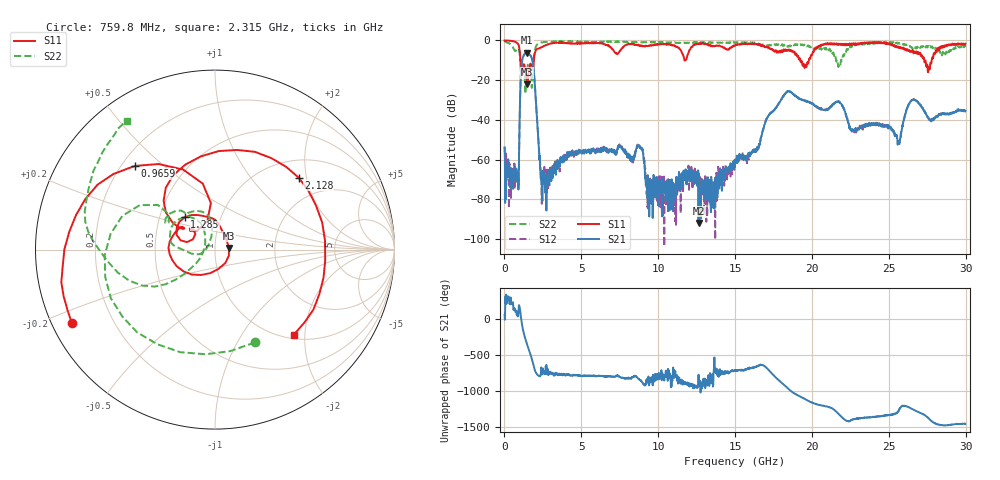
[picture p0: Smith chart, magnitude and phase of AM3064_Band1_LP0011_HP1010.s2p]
# Hz S DB R 50.0
!freq dBS11 angS11 dBS21 angS21 dBS12 angS12 dBS22 angS22
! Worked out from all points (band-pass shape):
!   1600 points, 10 MHz to 29.98 GHz, reference 50 ohm
!   highest |S21| = -6.19 dB at 1.453 GHz (marker M1); lowest = -92.0 dB at 12.62 GHz (marker M2)
!   |S21| within 3 dB of the highest: 1.175 GHz to 1.787 GHz (612 MHz wide, 41.3 % of centre)
!   lowest |S11| = -22.1 dB at 1.491 GHz (marker M3), VSWR 1.17, Z = 58.4 + j0.987 ohm
!   |S11| at or under -10 dB: 1.031 GHz to 1.914 GHz (882.9 MHz wide, 60 % of centre); 19.25 GHz to 19.81 GHz (557.6 MHz wide, 2.86 % of centre); 27.3 GHz to 27.79 GHz (490.7 MHz wide, 1.78 % of centre)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
!   |S22| runs from -26.9 to -0.2 dB; largest |S21 - S12| = 0.0086
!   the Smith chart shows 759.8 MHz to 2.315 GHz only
!   S11 on the Smith chart (normalised r, x): 759.8 MHz: 0.06, -0.24; 965.9 MHz: 0.25, +0.40; 1.285 GHz: 0.67, +0.26; 2.128 GHz: 1.39, +1.80; 2.315 GHz: 1.08, -1.76
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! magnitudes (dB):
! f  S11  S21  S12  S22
! 10 MHz  -0.1  -53.9  -53.5  -0.2
! 759.8 MHz  -0.9  -65.1  -65.3  -5.0
! 965.9 MHz  -3.8  -49.3  -49.2  -5.2
! 1.285 GHz  -12.2  -7.2  -7.1  -14.2
! 1.453 GHz  -20.0  -6.2  -6.1  -15.9
! 1.491 GHz  -22.1  -6.3  -6.2  -13.5
! 1.828 GHz  -13.4  -10.5  -10.4  -17.7
! 2.128 GHz  -4.2  -40.6  -40.2  -2.2
! 2.315 GHz  -3.8  -64.8  -59.9  -1.2
! 5.015 GHz  -1.5  -56.2  -56.3  -0.8
! 8.801 GHz  -2.7  -53.5  -54.0  -0.9
! 9.326 GHz  -2.9  -67.8  -73.4  -1.0
! 10 GHz  -2.0  -70.9  -79.6  -0.9
! 12.62 GHz  -1.6  -92.0  -70.1  -0.9
! 15 GHz  -2.5  -62.1  -60.8  -1.4
! 18.34 GHz  -5.3  -26.0  -26.1  -2.7
! 19.99 GHz  -7.5  -31.7  -31.8  -3.4
! 25 GHz  -1.5  -43.6  -42.6  -1.0
! 25.67 GHz  -3.8  -52.0  -50.5  -1.4
! 26.59 GHz  -5.8  -29.9  -30.0  -3.5
! 27.56 GHz  -15.8  -39.2  -38.5  -2.9
! 29.98 GHz  -1.7  -35.4  -35.4  -3.3
